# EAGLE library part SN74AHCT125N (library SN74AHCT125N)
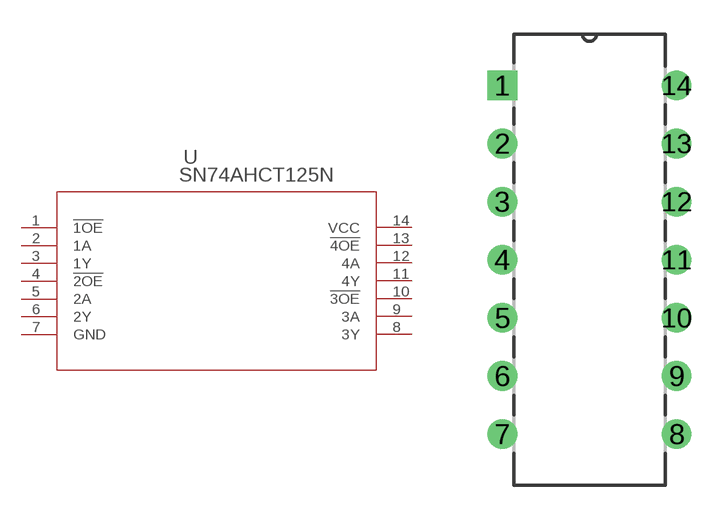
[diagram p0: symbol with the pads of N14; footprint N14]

Designator prefix U

## SN74AHCT125N (COPYRIGHT: Copyright (C) 2022 Ultra Librarian. All rights reserved.; MANUFACTURER_PART_NUMBER: SN74AHCT125N; MFR_NAME: Texas Instruments)  [N14]
1  !1OE  in
2  1A  in
3  1Y  pas
4  !2OE  in
5  2A  in
6  2Y  pas
7  GND  pwr
8  3Y  pas
9  3A  in
10  !3OE  in
11  4Y  pas
12  4A  in
13  !4OE  in
14  VCC  pwr

## Footprint N14 (pad centres in mm)
drill 0.787 pad 1.295 square: 1 -7.62,15.24
drill 0.787 pad 1.295: 2 -7.62,12.7; 3 -7.62,10.16; 4 -7.62,7.62; 5 -7.62,5.08; 6 -7.62,2.54; 7 -7.62,0; 8 0,0; 9 0,2.54; 10 0,5.08; 11 0,7.62; 12 0,10.16; 13 0,12.7; 14 0,15.24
